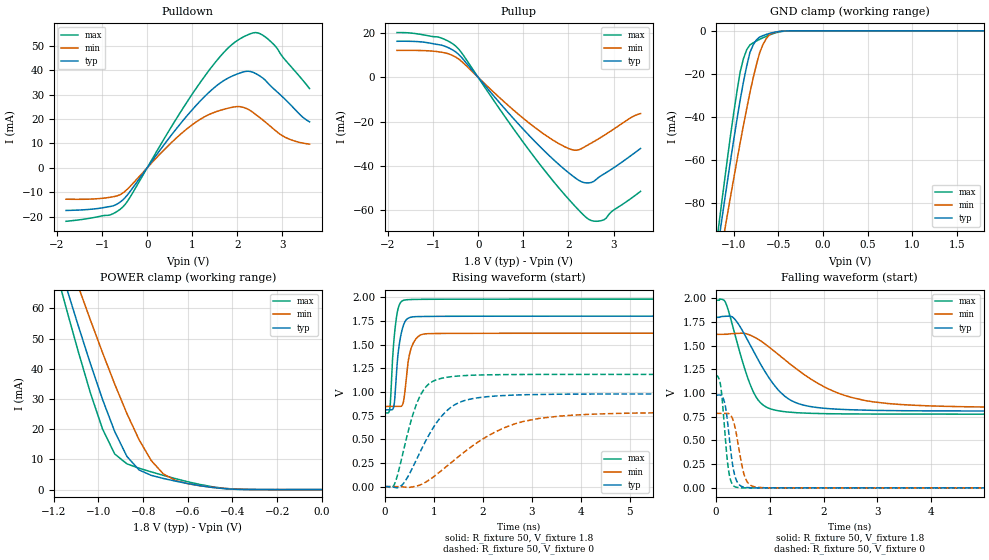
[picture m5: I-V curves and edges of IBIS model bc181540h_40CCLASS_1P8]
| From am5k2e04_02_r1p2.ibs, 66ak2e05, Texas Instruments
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|   Model Cell bc181540h_40CCLASS_1P8
|bc181540h_40CCLASS_1P8
[Model]   bc181540h_40CCLASS_1P8
Model_type   I/O
Polarity   Non-Inverting
Enable   Active-Low
Vinl =  0.63
Vinh =  1.17
Cref =  15.0000pF
Rref =  100.0000M
Vref =  0V
Vmeas =  0.9
C_comp   1.16613p   0.553312p   1.16742p
[Model Spec]
Vinl   0.63   0.567   0.693
Vinh   1.17   1.053   1.287
[Temperature Range]   25   125   -40
[Voltage Range]   1.8   1.62   1.98
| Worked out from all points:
|   slope of the pulldown table from 0 to 0.27 V, typ, clamps not added: 39.2 ohm
|   slope of the pullup table from 0 to 0.27 V, typ, clamps not added: 40.9 ohm
|   GND clamp passes 1 mA (typ) near -0.58 V on its own axis
|   POWER clamp passes 1 mA (typ) near -0.52 V on its own axis
|   rising waveform, R_fixture 50, V_fixture 1.8: 20-80 % time 114ps typ, 130ps min, 98.1ps max; typ from 0.811 V to 1.8 V
|   rising waveform, R_fixture 50, V_fixture 0: 20-80 % time 668ps typ, 1.35ns min, 396ps max; typ from 0 V to 0.979 V
|   falling waveform, R_fixture 50, V_fixture 1.8: 20-80 % time 651ps typ, 1.23ns min, 394ps max; typ from 1.8 V to 0.811 V
|   falling waveform, R_fixture 50, V_fixture 0: 20-80 % time 127ps typ, 156ps min, 107ps max; typ from 0.979 V to 0 V
[POWER_clamp]
|   voltage   I(typ)   I(min)   I(max)
-1.8V     235.9mA    223mA      250.7mA
-1.164V   71.87mA    82.65mA    65.36mA
-1.127V   63.07mA    75mA       55.51mA
-1.073V   50.17mA    63.68mA    41.25mA
-981.8mV  29.88mA    45.37mA    20.07mA
-927.3mV  19.23mA    34.95mA    11.8mA
-872.7mV  11mA       25.21mA    8.54mA
-818.2mV  6.508mA    16.53mA    7.086mA
-763.6mV  4.722mA    9.611mA    5.869mA
-709.1mV  3.682mA    5.172mA    4.713mA
-490.9mV  715.9uA    765.4uA    948.8uA
0V        973.6pA    18.39nA    2.408nA
[Pulldown]
|   voltage   I(typ)   I(min)   I(max)
-1.8V     -17.49mA   -12.88mA   -21.94mA
-818.2mV  -15.86mA   -12.08mA   -19.3mA
-545.5mV  -13.25mA   -10.42mA   -16.15mA
490.9mV   12.32mA    9.498mA    15.44mA
1.036V    24.59mA    18.17mA    31.25mA
1.691V    35.67mA    23.94mA    47.16mA
2.127V    39.29mA    24.81mA    53.62mA
2.4V      38.7mA     21.96mA    55.46mA
2.618V    35.92mA    18.78mA    53.67mA
2.836V    31.87mA    15.36mA    50.01mA
3.055V    28.14mA    12.57mA    44.34mA
3.6V      18.85mA    9.7mA      32.48mA
[Pullup]
|   voltage   I(typ)   I(min)   I(max)
-1.8V     16.38mA    12.23mA    20.34mA
-872.7mV  14.84mA    11.61mA    18.24mA
-490.9mV  11.44mA    9.116mA    14.06mA
818.2mV   -19.46mA   -15.43mA   -24.31mA
1.582V    -35.6mA    -27.44mA   -44.98mA
2.127V    -45.2mA    -32.99mA   -57.98mA
2.291V    -47.33mA   -32.3mA    -61.49mA
2.455V    -47.84mA   -30.39mA   -64.41mA
2.618V    -46.24mA   -28.46mA   -65.26mA
2.782V    -43.87mA   -26.41mA   -64.63mA
2.945V    -41.78mA   -24.25mA   -61.08mA
3.6V      -32.22mA   -16.39mA   -51.67mA
[GND_clamp]
|   voltage   I(typ)   I(min)   I(max)
-1.8V     -286.5mA   -268.3mA   -306.4mA
-1.182V   -101.5mA   -112.2mA   -95.12mA
-1.145V   -91mA      -103.2mA   -83.18mA
-1.109V   -80.68mA   -94.46mA   -71.51mA
-1.073V   -70.47mA   -85.72mA   -60.02mA
-927.3mV  -31.93mA   -51.83mA   -19.01mA
-890.9mV  -23.7mA    -43.85mA   -12.93mA
-818.2mV  -10.01mA   -28.59mA   -6.521mA
-709.1mV  -2.875mA   -10.12mA   -3.938mA
-600mV    -1.201mA   -1.844mA   -1.918mA
-490.9mV  -279uA     -308.3uA   -510uA
1.8V      973.6pA    1.906uA    493.4pA
[Ramp]
| variable   typ   min   max
dV/dt_f   0.601158/0.65600409n   0.471798/1.2411975n   0.728394/0.39655242n
dV/dt_r  0.5952486/0.67264275n  0.4782252/1.360014n   0.7184568/0.39795612n
R_load = 50
[Rising Waveform]
R_fixture = 50
V_fixture = 1.8
V_fixture_min = 1.62
V_fixture_max = 1.98
|   time   V(typ)   V(min)   V(max)
0s        810.7mV    846.4mV    777.9mV
100.7ps   810.8mV    846.4mV    818.3mV
183.9ps   847.7mV    846.3mV    1.535V
286.7ps   1.473V     846.1mV    1.907V
369ps     1.686V     874.4mV    1.965V
424.3ps   1.753V     1.074V     1.972V
482.8ps   1.781V     1.34V      1.975V
556.9ps   1.792V     1.488V     1.976V
853.5ps   1.797V     1.614V     1.978V
16.75ns   1.8V       1.62V      1.98V
[Rising Waveform]
R_fixture = 50
V_fixture = 0
V_fixture_min = 0
V_fixture_max = 0
|   time   V(typ)   V(min)   V(max)
0s        0V         0V         0V
214.2ps   -9.624mV   0V         46.29mV
366.8ps   24.69mV    -3.152mV   348.6mV
553ps     185.6mV    -4.278mV   726.8mV
757.3ps   404.6mV    25.45mV    992.4mV
965ps     602.9mV    92.08mV    1.107V
1.312ns   822.1mV    235.5mV    1.158V
2.48ns    963.2mV    629.6mV    1.183V
3.739ns   976.4mV    751.2mV    1.185V
16.71ns   978.8mV    786.4mV    1.185V
[Falling Waveform]
R_fixture = 50
V_fixture = 1.8
V_fixture_min = 1.62
V_fixture_max = 1.98
|   time   V(typ)   V(min)   V(max)
0s        1.8V       1.62V      1.98V
183.4ps   1.811V     1.62V      1.953V
378ps     1.762V     1.63V      1.568V
596.8ps   1.55V      1.621V     1.153V
745.4ps   1.392V     1.582V     959.6mV
941ps     1.201V     1.507V     851.2mV
1.301ns   958.7mV    1.342V     801.9mV
2.276ns   829.7mV    998.6mV    781.1mV
3.52ns    813.8mV    876.4mV    778.3mV
16.75ns   810.7mV    846.4mV    777.9mV
[Falling Waveform]
R_fixture = 50
V_fixture = 0
V_fixture_min = 0
V_fixture_max = 0
|   time   V(typ)   V(min)   V(max)
0s        978.8mV    786.4mV    1.185V
95.2ps    976.5mV    786.4mV    1.059V
174.4ps   872.5mV    786.2mV    531.4mV
215.7ps   705.6mV    787.1mV    275.8mV
256.6ps   491.9mV    777.2mV    120.4mV
344.5ps   145.5mV    667.7mV    14.23mV
454.8ps   23.69mV    322.1mV    0V
589.1ps   2.972mV    57.95mV    0V
916.2ps   0V         0V         0V
16.71ns   0V         0V         0V
